FUNCTION "TOT_PEZZI" : VOID
TITLE =CONTAPEZZI
VERSION : 0.1

BEGIN
NETWORK
TITLE =CONTAPEZZI PRODOTTO

      UN    "rdo prodteller-1";
      R     M     19.3;

      U     "rdo prodteller-1";
      UN    M     19.3;
      SPBN  M001;
      L     "DB_TD_OP37".Count_tot_R;
      L     L#1;
      +D    ;
      T     "DB_TD_OP37".Count_tot_R;
      S     M     19.3;

M001: NOP   0;
      UN    E      5.7;
      R     M     19.2;

      U     E      5.7;
      UN    M     19.2;
      SPBN  M002;
      L     "DB_TD_OP37".Count_tot_R;
      L     L#1;
      +D    ;
      T     "DB_TD_OP37".Count_tot_R;
      S     M     19.2;
M002: NOP   0;

NETWORK
TITLE =PARTIAL AND TOTAL COUNTER
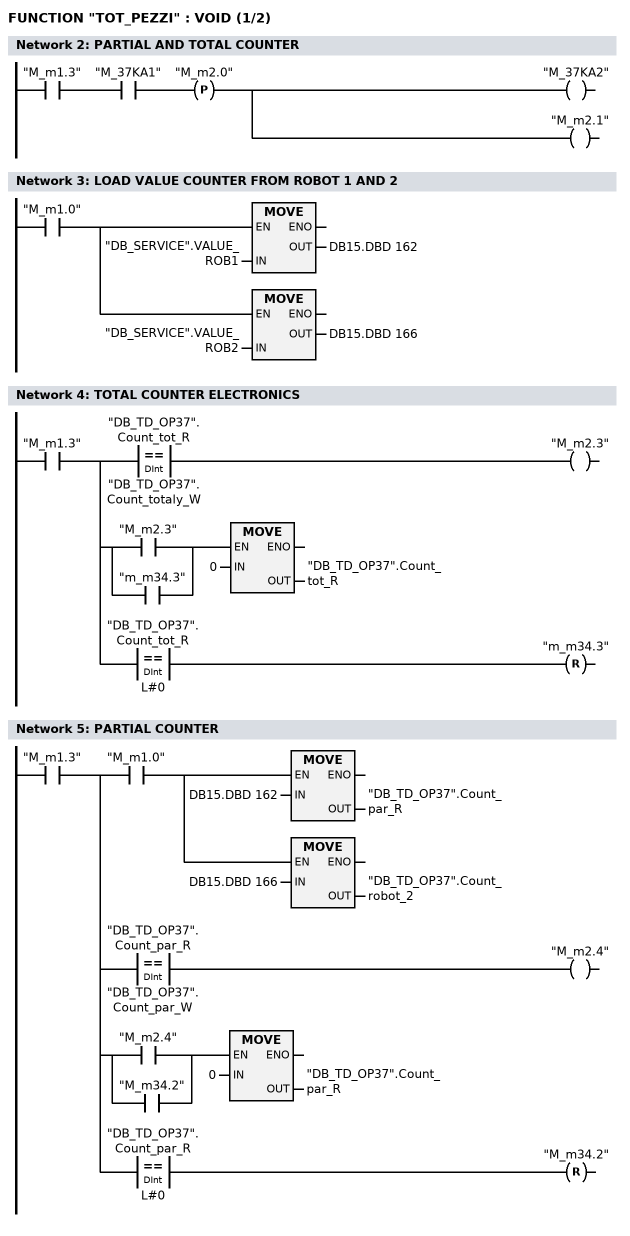
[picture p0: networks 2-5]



      U     "M_m1.3";
      U     "M_37KA1";
      FP    "M_m2.0";
      =     "M_37KA2";
      =     "M_m2.1";
NETWORK
TITLE =LOAD VALUE COUNTER FROM ROBOT 1 AND 2



      U     "M_m1.0";
      =     L      0.0;
      U     L      0.0;
      SPBNB _001;
      L     "DB_SERVICE".VALUE_ROB1;
      T     DB15.DBD  162;
_001: NOP   0;
      U     L      0.0;
      SPBNB _01c;
      L     "DB_SERVICE".VALUE_ROB2;
      T     DB15.DBD  166;
_01c: NOP   0;
NETWORK
TITLE =TOTAL COUNTER ELECTRONICS



      U     "M_m1.3";
      =     L      0.0;
      U     L      0.0;
      U(    ;
      L     "DB_TD_OP37".Count_tot_R;
      L     "DB_TD_OP37".Count_totaly_W;
      ==D   ;
      )     ;
      =     "M_m2.3";
      U     L      0.0;
      U(    ;
      O     "M_m2.3";
      O     "m_m34.3";
      )     ;
      SPBNB _01d;
      L     0;
      T     "DB_TD_OP37".Count_tot_R;
_01d: NOP   0;
      U     L      0.0;
      U(    ;
      L     "DB_TD_OP37".Count_tot_R;
      L     L#0;
      ==D   ;
      )     ;
      R     "m_m34.3";
NETWORK
TITLE =PARTIAL COUNTER



      U     "M_m1.3";
      =     L      0.0;
      U     L      0.0;
      U     "M_m1.0";
      =     L      0.1;
      U     L      0.1;
      SPBNB _01e;
      L     DB15.DBD  162;
      T     "DB_TD_OP37".Count_par_R;
_01e: NOP   0;
      U     L      0.1;
      SPBNB _01f;
      L     DB15.DBD  166;
      T     "DB_TD_OP37".Count_robot_2;
_01f: NOP   0;
      U     L      0.0;
      U(    ;
      L     "DB_TD_OP37".Count_par_R;
      L     "DB_TD_OP37".Count_par_W;
      ==D   ;
      )     ;
      =     "M_m2.4";
      U     L      0.0;
      U(    ;
      O     "M_m2.4";
      O     "M_m34.2";
      )     ;
      SPBNB _020;
      L     0;
      T     "DB_TD_OP37".Count_par_R;
_020: NOP   0;
      U     L      0.0;
      U(    ;
      L     "DB_TD_OP37".Count_par_R;
      L     L#0;
      ==D   ;
      )     ;
      R     "M_m34.2";
NETWORK
TITLE =MAINTENANCE COUNTER
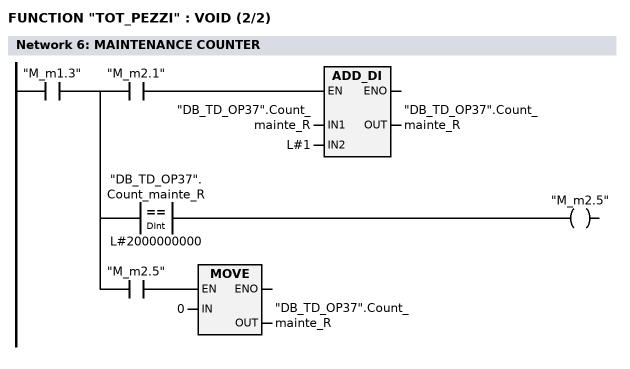
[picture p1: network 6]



      U     "M_m1.3";
      =     L      0.0;
      U     L      0.0;
      U     "M_m2.1";
      SPBNB _021;
      L     "DB_TD_OP37".Count_mainte_R;
      L     L#1;
      +D    ;
      T     "DB_TD_OP37".Count_mainte_R;
_021: NOP   0;
      U     L      0.0;
      U(    ;
      L     "DB_TD_OP37".Count_mainte_R;
      L     L#2000000000;
      ==D   ;
      )     ;
      =     "M_m2.5";
      U     L      0.0;
      U     "M_m2.5";
      SPBNB _022;
      L     0;
      T     "DB_TD_OP37".Count_mainte_R;
_022: NOP   0;
NETWORK
TITLE =MAINTENANCE COUNTER



END_FUNCTION

